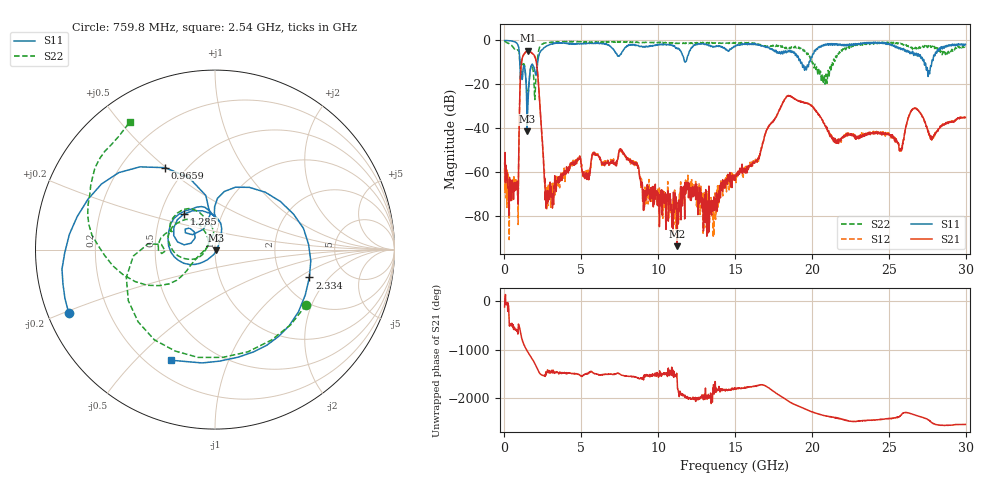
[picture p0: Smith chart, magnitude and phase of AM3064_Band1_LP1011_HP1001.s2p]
# Hz S DB R 50.0
!freq dBS11 angS11 dBS21 angS21 dBS12 angS12 dBS22 angS22
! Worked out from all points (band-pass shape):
!   1600 points, 10 MHz to 29.98 GHz, reference 50 ohm
!   highest |S21| = -4.77 dB at 1.528 GHz (marker M1); lowest = -93.9 dB at 11.24 GHz (marker M2)
!   |S21| within 3 dB of the highest: 1.172 GHz to 1.997 GHz (825.3 MHz wide, 52.1 % of centre)
!   lowest |S11| = -41.6 dB at 1.472 GHz (marker M3), VSWR 1.02, Z = 50.7 - j0.453 ohm
!   |S11| at or under -10 dB: 1.002 GHz to 2.161 GHz (1.159 GHz wide, 73.3 % of centre); 19.26 GHz to 19.81 GHz (553.5 MHz wide, 2.83 % of centre); 27.3 GHz to 27.79 GHz (494.8 MHz wide, 1.8 % of centre)
!   |S22| runs from -27.0 to -0.3 dB; largest |S21 - S12| = 0.0071
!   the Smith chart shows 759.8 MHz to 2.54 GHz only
!   S11 on the Smith chart (normalised r, x): 759.8 MHz: 0.06, -0.21; 965.9 MHz: 0.39, +0.50; 1.285 GHz: 0.66, +0.28; 2.334 GHz: 2.81, -1.25; 2.54 GHz: 0.29, -0.64
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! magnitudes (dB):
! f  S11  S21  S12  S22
! 10 MHz  0.0  -56.1  -58.2  -0.3
! 759.8 MHz  -1.0  -65.1  -63.7  -4.5
! 965.9 MHz  -5.5  -35.9  -36.0  -6.8
! 1.285 GHz  -11.6  -6.2  -6.1  -10.9
! 1.472 GHz  -41.6  -4.9  -4.8  -23.6
! 1.528 GHz  -29.2  -4.8  -4.7  -25.9
! 2.034 GHz  -15.6  -8.7  -8.5  -18.0
! 2.334 GHz  -5.2  -32.7  -32.7  -2.5
! 2.54 GHz  -3.6  -55.0  -55.0  -1.4
! 2.803 GHz  -2.4  -69.1  -73.0  -1.0
! 5.015 GHz  -1.4  -57.3  -56.5  -0.8
! 7.62 GHz  -5.7  -49.9  -50.0  -0.7
! 10 GHz  -2.0  -73.3  -69.4  -1.0
! 11.24 GHz  -3.6  -93.9  -77.3  -1.3
! 15 GHz  -2.7  -62.9  -61.9  -1.4
! 18.34 GHz  -5.6  -25.8  -25.8  -3.5
! 19.99 GHz  -7.8  -30.0  -30.0  -9.3
! 21.55 GHz  -1.9  -46.4  -46.0  -7.2
! 25 GHz  -1.4  -42.5  -42.1  -1.1
! 26.68 GHz  -5.8  -31.1  -30.9  -3.7
! 27.58 GHz  -14.6  -41.5  -42.3  -2.4
! 29.98 GHz  -1.8  -35.1  -35.1  -3.1
